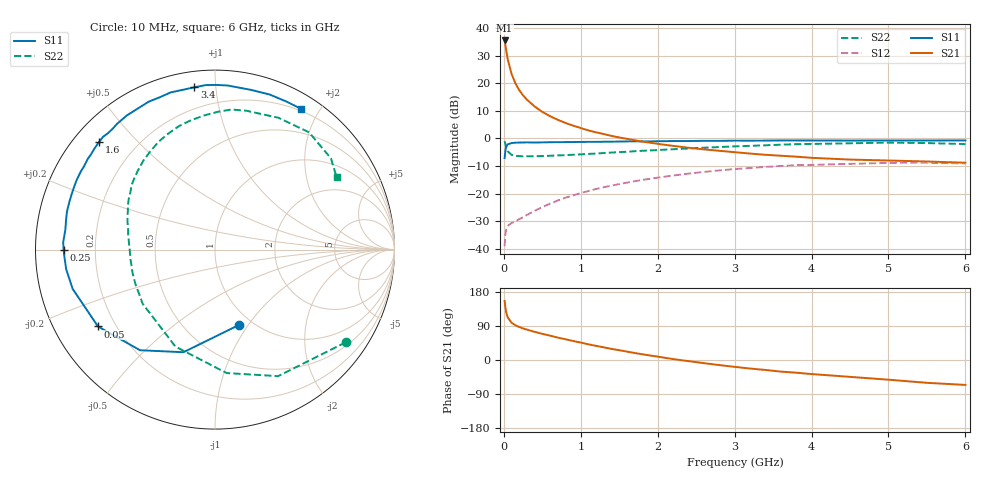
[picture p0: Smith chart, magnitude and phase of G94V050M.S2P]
! SIEMENS Small Signal Semiconductors
! BFG235
! Si NPN RF Bipolar Junction Transistor in SOT223
! VCE = 4 V  IC = 50 mA
! Common Emitter S-Parameters:  July  1994
# GHz  S  MA  R  50
!  f  S11  S21  S12  S22
! GHz  MAG  ANG  MAG  ANG  MAG  ANG  MAG  ANG
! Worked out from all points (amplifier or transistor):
!   40 points, 10 MHz to 6 GHz, reference 50 ohm
!   highest |S21| = 35.5 dB at 10 MHz (marker M1)
!   |S21| within 3 dB of that: start of sweep to 27.29 MHz
!   unconditionally stable (mu >= 1): 487 MHz to 1.346 GHz
!   at 200 MHz: K = 0.68, MSG = 23.4 dB, |S12| = -29.3 dB
!   at 1.5 GHz: K = 0.98, MSG = 8.4 dB, |S12| = -16.6 dB
!   at 6 GHz: K = 0.92, MSG = 0.1 dB, |S12| = -9.1 dB
!   S11 on the Smith chart (normalised r, x): 10 MHz: 0.87, -0.91; 50 MHz: 0.13, -0.29; 250 MHz: 0.08, -0.00; 1.6 GHz: 0.07, +0.39; 3.4 GHz: 0.08, +0.88; 6 GHz: 0.18, +1.77
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0.01  0.4405 -72.2  59.71 156.2  0.0111 68.0  0.8932 -35.3
0.02  0.5982 -107.1  49.07 138.5  0.0182 51.6  0.7879 -63.5
0.03  0.6992 -126.7  39.99 126.3  0.0221 43.1  0.6909 -84.6
0.05  0.7801 -146.7  27.5 112.5  0.0258 32.8  0.5836 -112.2
0.1  0.8228 -164.6  14.8 98.5  0.0292 30.0  0.5033 -143.2
0.15  0.8363 -172.5  9.982 91.7  0.0312 34.1  0.4829 -156.7
0.2  0.8393 -176.6  7.489 87.1  0.0343 37.1  0.4774 -164.2
0.25  0.8435 -180.0  6.035 83.3  0.0373 40.7  0.4737 -169.3
0.3  0.8468 177.3  5.041 80.2  0.0408 43.7  0.4737 -173.2
0.4  0.841 172.4  3.793 74.3  0.0486 47.9  0.4746 -178.7
0.5  0.8465 168.5  3.025 69.0  0.0567 50.9  0.4789 177.0
0.6  0.8518 165.4  2.528 64.3  0.0655 52.2  0.4841 173.4
0.7  0.8539 161.8  2.178 59.2  0.0747 52.9  0.4912 170.1
0.9  0.8588 156.3  1.706 50.2  0.0926 51.9  0.5049 164.4
1.1  0.865 149.9  1.394 41.3  0.1112 50.1  0.5228 158.7
1.6  0.881 137.3  0.983 22.2  0.1576 42.1  0.5719 145.3
2.2  0.8944 123.3  0.731 2.4  0.2121 29.8  0.6363 128.9
3.2  0.9082 101.5  0.531 -22.5  0.291 6.2  0.732 100.8
3.4  0.9115 97.2  0.504 -26.3  0.3035 1.3  0.7495 94.8
4.5  0.9122 77.4  0.413 -44.5  0.345 -24.7  0.8151 64.3
5.5  0.9158 64.3  0.381 -60.2  0.3617 -47.0  0.8222 38.2
6  0.9193 58.5  0.362 -65.8  0.351 -55.1  0.7887 30.8
